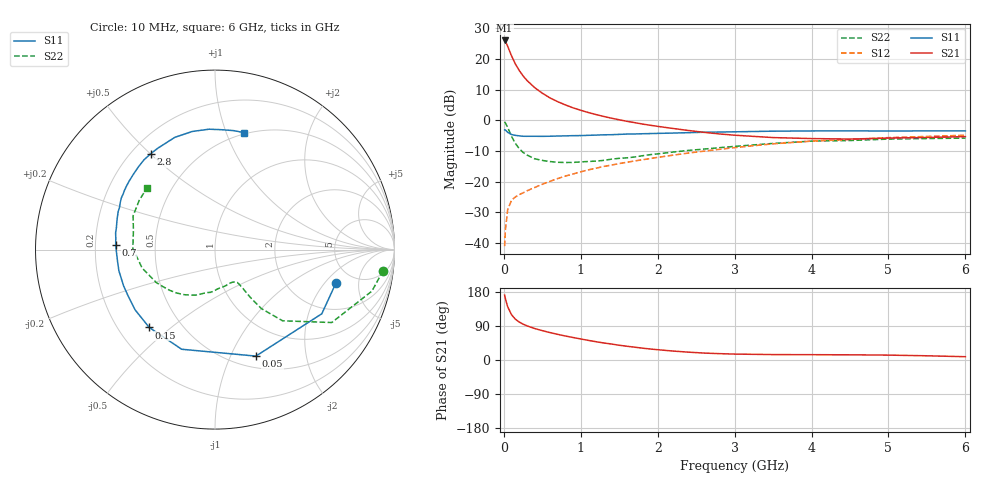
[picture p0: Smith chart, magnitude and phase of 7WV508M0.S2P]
! Infineon Technologies  Discrete & RF Semiconductors
! BFS17W
! Si NPN RF Bipolar Junction Transistor in SOT323
! VCE = 0.5 V  IC = 8 mA
! Common Emitter S-Parameters:  August  1999
# GHz  S  MA  R  50
!  f  S11  S21  S12  S22
! GHz  MAG  ANG  MAG  ANG  MAG  ANG  MAG  ANG
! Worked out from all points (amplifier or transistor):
!   36 points, 10 MHz to 6 GHz, reference 50 ohm
!   highest |S21| = 26.1 dB at 10 MHz (marker M1)
!   |S21| within 3 dB of that: start of sweep to 67.53 MHz
!   unconditionally stable (mu >= 1): 282.1 MHz to end of sweep
!   at 250 MHz: K = 0.93, MSG = 19.1 dB, |S12| = -23.7 dB
!   at 1.4 GHz: K = 1.54, MAG = 3.3 dB, |S12| = -14.6 dB
!   at 6 GHz: K = 1.15, MAG = -2.6 dB, |S12| = -4.9 dB
!   S11 on the Smith chart (normalised r, x): 10 MHz: 3.62, -2.64; 50 MHz: 0.63, -1.25; 150 MHz: 0.33, -0.42; 700 MHz: 0.29, +0.02; 2.8 GHz: 0.28, +0.50; 6 GHz: 0.49, +1.15
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0.01  0.699 -15.5  20.13 171.4  0.0088 80.1  0.9442 -7.1
0.02  0.6942 -31.0  19.57 161.9  0.016 77.1  0.9045 -14.8
0.05  0.6356 -69.0  16.17 140.4  0.0347 58.5  0.7669 -32.0
0.1  0.5854 -108.5  11.28 119.4  0.0495 46.3  0.5468 -46.5
0.15  0.5677 -130.2  8.306 107.6  0.0561 41.4  0.4183 -51.8
0.2  0.5575 -143.0  6.508 100.1  0.0612 41.7  0.3461 -53.3
0.25  0.5486 -151.9  5.318 94.6  0.0653 41.9  0.2985 -53.9
0.3  0.5479 -158.3  4.487 90.3  0.0706 44.0  0.2716 -54.2
0.4  0.5483 -167.6  3.421 83.1  0.0798 46.8  0.2355 -55.1
0.5  0.547 -173.7  2.769 77.5  0.0903 49.5  0.2213 -55.8
0.6  0.5492 -178.5  2.319 72.3  0.1009 51.5  0.2119 -58.1
0.7  0.5539 177.4  2.015 67.7  0.1117 52.9  0.2062 -61.7
0.9  0.5617 170.4  1.597 59.4  0.1328 54.2  0.2051 -69.6
1.1  0.5686 164.1  1.338 51.7  0.1551 54.7  0.2127 -78.2
1.3  0.5797 158.4  1.154 44.9  0.1764 54.5  0.2219 -87.7
1.6  0.5962 151.0  0.963 36.3  0.2064 54.0  0.2437 -100.6
2.2  0.6188 137.3  0.735 23.6  0.2697 52.0  0.3028 -123.8
2.8  0.6431 123.9  0.599 16.8  0.3353 48.0  0.3566 -144.8
3.5  0.6643 109.7  0.522 14.3  0.4128 41.1  0.4191 -165.9
4.5  0.6716 92.8  0.494 13.7  0.4858 29.5  0.4671 166.6
5.5  0.6711 80.9  0.524 11.1  0.5448 20.0  0.5035 147.0
6  0.6711 76.3  0.542 8.7  0.5705 15.2  0.5116 138.0
